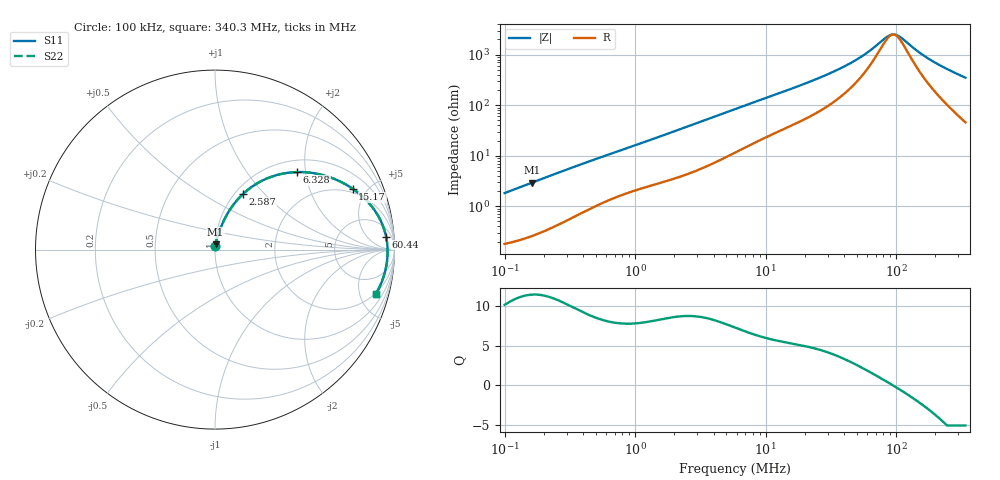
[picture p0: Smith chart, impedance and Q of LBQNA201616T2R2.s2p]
! LBQNA201616T2R2  S-PARAMETER MODEL  ( General Type )
! Model Generated by TAIYO YUDEN Corporation (http://www.ty-top.com)
! Version 1.0
! TAIYO YUDEN Control No. 191025NI43SB-FBB
! Copyright(c) 2019 TAIYO YUDEN CO.,LTD. All Rights Reserved.
! Product Description (link to TY-COMPAS)
! https://ds.yuden.co.jp/TYCOMPAS/or/detail?pn=LBQNA201616T2R2M&u=M
! Products Name : Inductors
! Characteristics :
!  Inductance : 2.2 uH , SRF(min) : 70 MHz , DC Resistance(max) : 0.169 Ohm
!  Rated Current : Saturation :510 mA , Temp Rise : 600 mA (20 degC)
!  Case Size : 2.0 x 1.6 / 0.079 x 0.063 [mm/inch] , Thickness : 1.6 / 0.063 [mm/inch]
!  (Conditions: Temperature = 25 degC , DC Bias Current/Voltage = 0A / 0V)
! External Node Assignments :
!  1  o---GGG---o  2
! GND o---------o GND
! Frequency Range : 0.1MHz  -  340.31115MHz  [ 402 STEP ]
# MHz S RI R 50
! Freq[MHz].  S11 Real  S11 Imag  S21 Real  S21 Imag  S12 Real  S12 Imag  S22 Real  S22 Imag
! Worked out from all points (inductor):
!   401 points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, 100 kHz to 340.3 MHz, reference 50 ohm
!   read as one part in series: L = 2.88 uH near 104.2 kHz
!   highest Q = 11.4 at 162.9 kHz (marker M1), where L = 2.87 uH
!   self-resonance near 95.07 MHz
!   S11 on the Smith chart (normalised r, x): 100 kHz: 1.00, +0.04; 2.587 MHz: 1.09, +0.77; 6.328 MHz: 1.26, +1.80; 15.17 MHz: 1.75, +4.01; 60.44 MHz: 12, +19; 340.3 MHz: 1.92, -6.95
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0.1  0.00212 0.0181  0.9979 -0.0181  0.9979 -0.0181  0.00212 0.0181
0.162897  0.00344 0.0292  0.9966 -0.0292  0.9966 -0.0292  0.00344 0.0292
0.390471  0.0118 0.0668  0.9882 -0.0668  0.9882 -0.0668  0.0118 0.0668
0.811817  0.0331 0.1257  0.9669 -0.1257  0.9669 -0.1257  0.0331 0.1257
1.524679  0.0758 0.2108  0.9242 -0.2108  0.9242 -0.2108  0.0758 0.2108
2.586726  0.1576 0.3114  0.8424 -0.3114  0.8424 -0.3114  0.1576 0.3114
3.806401  0.2639 0.3846  0.7361 -0.3846  0.7361 -0.3846  0.2639 0.3846
5.953437  0.4327 0.4308  0.5673 -0.4308  0.5673 -0.4308  0.4327 0.4308
6.32786  0.4575 0.4321  0.5425 -0.4321  0.5425 -0.4321  0.4575 0.4321
9.311528  0.6098 0.4126  0.3902 -0.4126  0.3902 -0.4126  0.6098 0.4126
15.16818  0.7669 0.339  0.2331 -0.339  0.2331 -0.339  0.7669 0.339
22.77862  0.8584 0.2584  0.1416 -0.2584  0.1416 -0.2584  0.8584 0.2584
39.43928  0.9289 0.1485  0.0711 -0.1485  0.0711 -0.1485  0.9289 0.1485
49.32369  0.9441 0.1076  0.0559 -0.1076  0.0559 -0.1076  0.9441 0.1076
60.4439  0.9531 0.0727  0.0469 -0.0727  0.0469 -0.0727  0.9531 0.0727
88.94399  0.9613 0.0105  0.0387 -0.0105  0.0387 -0.0105  0.9613 0.0105
96.47957  0.9617 -0.00233  0.0383 0.00233  0.0383 0.00233  0.9617 -0.00233
104.6536  0.9618 -0.0152  0.0382 0.0152  0.0382 0.0152  0.9618 -0.0152
147.8628  0.9575 -0.072  0.0425 0.072  0.0425 0.072  0.9575 -0.072
181.199  0.951 -0.1083  0.049 0.1083  0.049 0.1083  0.951 -0.1083
245.8109  0.9329 -0.1694  0.0671 0.1694  0.0671 0.1694  0.9329 -0.1694
340.3111  0.8972 -0.2448  0.1028 0.2448  0.1028 0.2448  0.8972 -0.2448
